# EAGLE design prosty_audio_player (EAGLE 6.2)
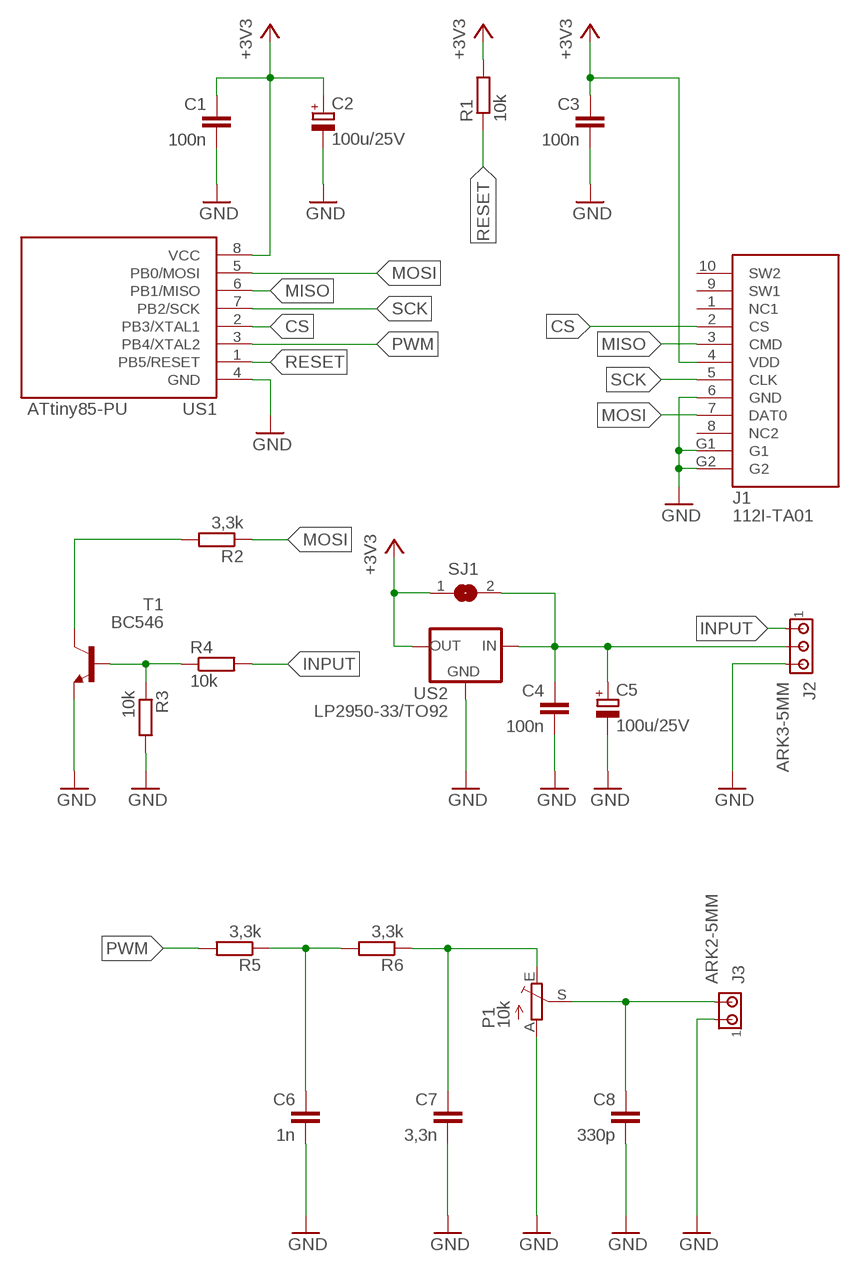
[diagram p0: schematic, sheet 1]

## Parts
C1  100n  C-EU050-025X075  [C050-025X075]
C2  100u/25V  CPOL-EUE2.5-5  [E2,5-5]
C3  100n  C-EU050-025X075  [C050-025X075]
C4  100n  C-EU050-025X075  [C050-025X075]
C5  100u/25V  CPOL-EUE2.5-5  [E2,5-5]
C6  1n  C-EU050-025X075  [C050-025X075]
C7  3,3n  C-EU050-025X075  [C050-025X075]
C8  330p  C-EU050-025X075  [C050-025X075]
J1  112I-TA01  MICRO-SD-112I-TA01-B-2  [MICRO-SD-112I-TA01-B-2]
J2  ARK3-5MM  [3PIN-5MM]
J3  ARK2-5MM  [2PIN-5MM]
P1  10k  TRIM_EU-CA6V  [CA6V]
R1  10k  R-EU_0207/7  [0207/7]
R2  3,3k  R-EU_0207/7  [0207/7]
R3  10k  R-EU_0207/7  [0207/7]
R4  10k  R-EU_0207/7  [0207/7]
R5  3,3k  R-EU_0207/7  [0207/7]
R6  3,3k  R-EU_0207/7  [0207/7]
SJ1  SJ  [SJ]
T1  BC546  BC546A  [TO92-EBC]
US1  ATtiny85-PU  ATTINY25-DIL8  [DIL08]
US2  LP2950-33/TO92  78LXX  [78LXX]

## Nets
+3V3: C1.1 C2.+ C3.1 J1.4(VDD) R1.2 SJ1.1 US1.8(VCC) US2.OUT
CS: J1.2(CS) US1.2(PB3/XTAL1)
GND: C1.2 C2.- C3.2 C4.2 C5.- C6.2 C7.2 C8.2 J1.6(GND) J1.G1 J1.G2 J2.P$3 J3.P$1 P1.A R3.2 T1.E US1.4(GND) US2.GND
INPUT: J2.P$1 R4.2
MISO: J1.3(CMD) US1.6(PB1/MISO)
MOSI: J1.7(DAT0) R2.1 US1.5(PB0/MOSI)
N$1: R2.2 T1.C
N$2: R3.1 R4.1 T1.B
N$3: C6.1 R5.1 R6.2
N$4: C7.1 P1.E R6.1
N$5: C8.1 J3.P$2 P1.S
N$6: C4.1 C5.+ J2.P$2 SJ1.2 US2.IN
PWM: R5.2 US1.3(PB4/XTAL2)
RESET: R1.1 US1.1(PB5/RESET)
SCK: J1.5(CLK) US1.7(PB2/SCK)
Unconnected: J1.1(NC1) J1.8(NC2) J1.9(SW1) J1.10(SW2)

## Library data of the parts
C1 C3 C4 C6-C8 = rcl:C-EU: CAPACITOR, European symbol
C2 C5 = rcl:CPOL-EU: POLARIZED CAPACITOR, European symbol
J1 = inne_futrzak:MICRO-SD-112I-TA01-B-2
J2 = zlacza_futrzak:ARK3: ARK 3 Raster 5mm i 3,5mm
J3 = zlacza_futrzak:ARK2: ARK 2
P1 = pot:TRIM_EU-: POTENTIOMETER
R1-R6 = rcl:R-EU_: RESISTOR, European symbol
SJ1 = jumper:SJ: SMD solder JUMPER
T1 = transistor-npn:BC546*: NPN Transistor
US1 = scalaki_futrzak:ATTINY25
US2 = v-reg:78LXX: VOLTAGE REGULATOR

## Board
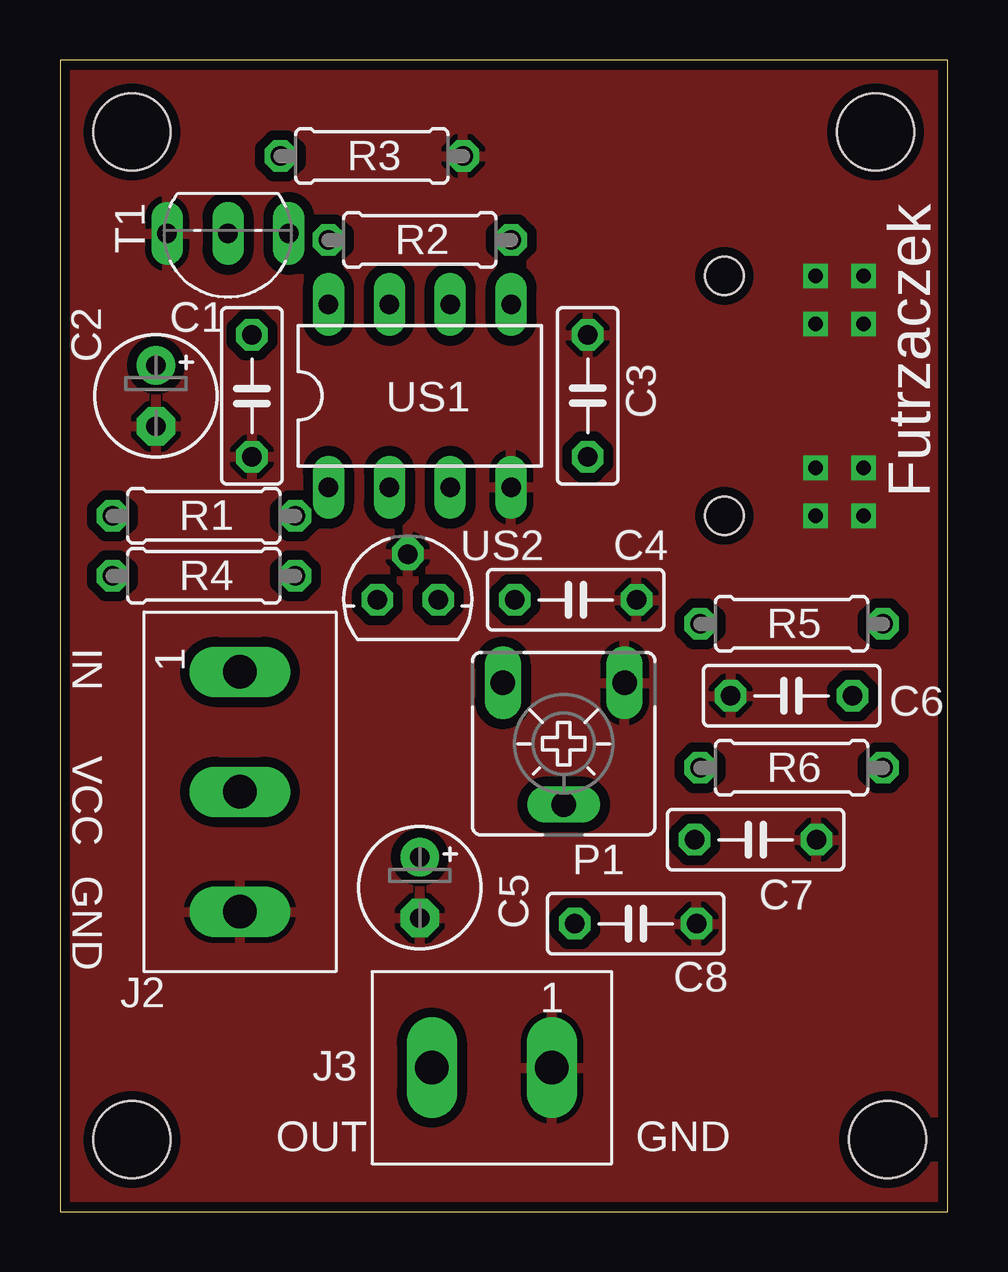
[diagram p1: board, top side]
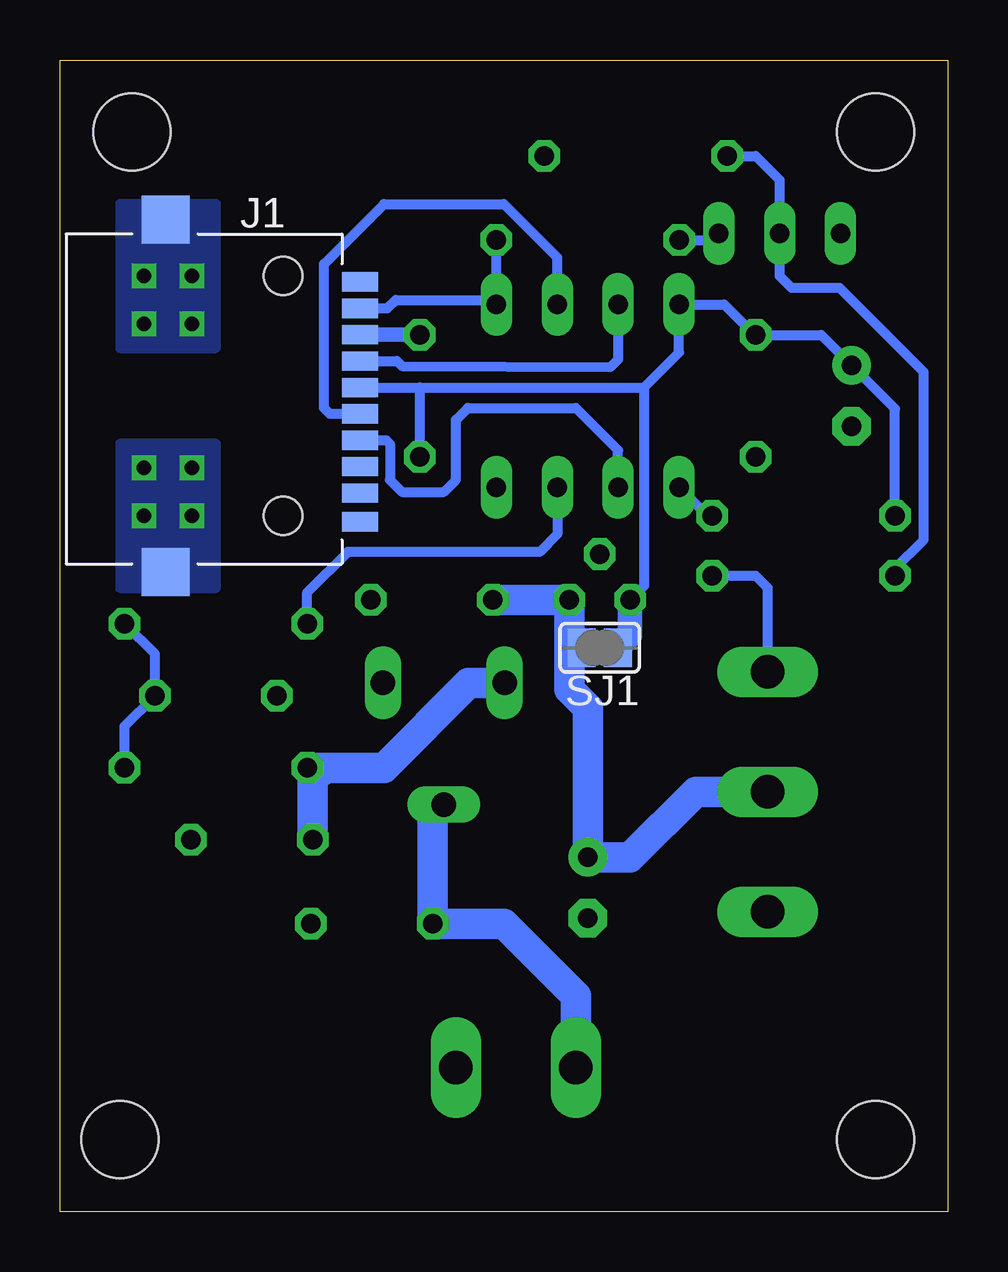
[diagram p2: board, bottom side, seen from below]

Size 37 x 48 mm. Coordinates in mm from the lower left corner, seen from the top.
Outline: 0,0 37,0 37,48 0,48 0,0
Copper layers (1*16): Top 0.035mm / dielectric 1.5mm / Bottom 0.035mm
Design rules: minimum track width 10mil, minimum drill 24mil, track to track 8mil, track to pad 8mil, pad to pad 8mil, via to via 8mil, smd to smd 8mil, copper to edge 10mil, drill to drill 8mil, minimum pad ring 10mil, minimum via ring 8mil, stop-mask expansion 4mil, vias tented up to drill 0mil, thermal gap 10mil
Holes 3.2 mm at 3,3 34.5,3 3,45 34,45

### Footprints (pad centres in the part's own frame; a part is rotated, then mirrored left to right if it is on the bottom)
C050-025X075 = drill 0.813 octagon: 1 -2.54,0; 2 2.54,0
E2,5-5 = drill 0.813 pad 1.6: + -1.27,0 | drill 0.813 pad 1.6 octagon: - 1.27,0
MICRO-SD-112I-TA01-B-2 = smd 0.8 x 1.5: 1 2.95,0; 2 1.85,0; 3 0.75,0; 4 -0.35,0; 5 -1.45,0; 6 -2.55,0; 7 -3.65,0; 8 -4.75,0; 9 5.25,0; 10 4.05,0 | smd 2 x 2: G1 -7.35,-8.1; G2 7.35,-8.1 | hole 1.6: -5,-3.2; 5,-3.2
3PIN-5MM = drill 1.4 long: P$1 -5,0; P$2 0,0; P$3 5,0
2PIN-5MM = drill 1.4 long: P$1 -2.5,0; P$2 2.5,0
CA6V = drill 1.016 long: A -2.54,-2.54; E 2.54,-2.54; S 0,2.54
0207/7 = drill 0.813 octagon: 1 -3.81,0; 2 3.81,0
SJ = smd 1.168 x 1.6: 1 -0.762,0; 2 0.762,0
TO92-EBC = drill 0.813 long: B 0,-1.27; C -2.54,-1.27; E 2.54,-1.27
DIL08 = drill 0.813 long: 1 -3.81,-3.81; 2 -1.27,-3.81; 3 1.27,-3.81; 4 3.81,-3.81; 5 3.81,3.81; 6 1.27,3.81; 7 -1.27,3.81; 8 -3.81,3.81
78LXX = drill 0.813 octagon: GND 0,1.905; IN 1.27,0; OUT -1.27,0

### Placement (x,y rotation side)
C1  8,34 270 top
C2  4,34 270 top
C3  22,34 90 top
C4  21.5,25.5 0 top
C5  15,13.5 270 top
C6  30.5,21.5 180 top
C7  29,15.5 0 top
C8  24,12 0 top
J1  24.5,34 270 bottom
J2  7.5,17.5 270 top
J3  18,6 180 top
P1  21,19.5 180 top
R1  6,29 180 top
R2  15,40.5 180 top
R3  13,44 0 top
R4  6,26.5 0 top
R5  30.5,24.5 180 top
R6  30.5,18.5 0 top
SJ1  14.5,23.5 180 bottom
T1  7,39.5 180 top
US1  15,34 0 top
US2  14.5,25.5 0 top

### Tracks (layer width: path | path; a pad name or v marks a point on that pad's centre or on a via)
+3V3
  Bottom 0.406: J1.4 22,34.35 | 22,34.35 12.65,34.35 | 12.65,34.35 11.19,35.81 US1.8 9.31,37.81 8.04,36.54 C1.1 5.27,36.54 C2.+ 2.19,33.46 R1.2 | C3.1 22,34.35 | 12.65,34.35 12.65,26.08 US2.OUT
  Bottom 1.016: US2.OUT 13.23,24.01 SJ1.1
CS
  Bottom 0.406: US1.2 13.73,31.73 15.5,33.5 20,33.5 20.5,33 20.5,30.5 21,30 22.75,30 23.25,30.5 23.25,32 23.4,32.15 J1.2
GND  (via drill 0.6)
  Bottom 0.406: 4.5,40.73 T1.E
  Bottom 0.61: J1.6 C3.2
  other vias: 31.5,39 33.5,39 31.5,37 33.5,37 31.5,29 33.5,29 33.5,31 31.5,31
  pour Bottom (isolate 0.406, no thermals): 30.5,42 34.5,42 34.5,36 30.5,36
  pour Bottom (isolate 0.406, no thermals): 30.5,32 34.5,32 34.5,26 30.5,26
  pour Top (isolate 0.406): 0,0 37,0 37,48 0,48
INPUT
  Bottom 0.406: J2.P$1 7.5,26 8,26.5 R4.2
MISO
  Bottom 0.406: J1.3 25.75,33.25 26,33.5 26,39.5 23.5,42 18.5,42 16.27,39.77 US1.6
MOSI
  Bottom 0.406: J1.7 23.35,37.65 23,38 19,38 US1.5 R2.1
N$1
  Bottom 0.406: R2.2 9.81,40.5 T1.C
N$2
  Bottom 0.406: R3.1 8,44 7,43 T1.B 7,39 6.5,38.5 4.5,38.5 1,35 1,28 2.19,26.81 R4.1
N$3
  Bottom 0.406: R5.1 33.04,23.23 C6.1 34.31,20.23 R6.2
N$4
  Bottom 1.27: R6.1 26,18.5 | 26,18.5 23.5,18.5 19.96,22.04 P1.E | C7.1 26.46,18.04 26,18.5
N$5
  Bottom 1.27: J3.P$2 15.5,9 18.5,12 C8.1 21.46,16.5 P1.S
N$6
  Bottom 1.016: SJ1.2 15.77,23.5
  Bottom 1.27: J2.P$2 10.5,17.5 13.23,14.77 C5.+ 15,21 15.77,21.77 15.77,23.5 US2.IN C4.1
PWM
  Bottom 0.406: US1.3 16.27,28.23 17,27.5 25,27.5 26.69,25.81 R5.2
RESET
  Bottom 0.406: R1.1 10,29 US1.1
SCK
  Bottom 0.406: J1.5 22.95,35.45 22.75,35.25 14.05,35.2 13.73,35.52 US1.7

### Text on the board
tPlace: Futrzaczek | IN | VCC | GND | OUT | GND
